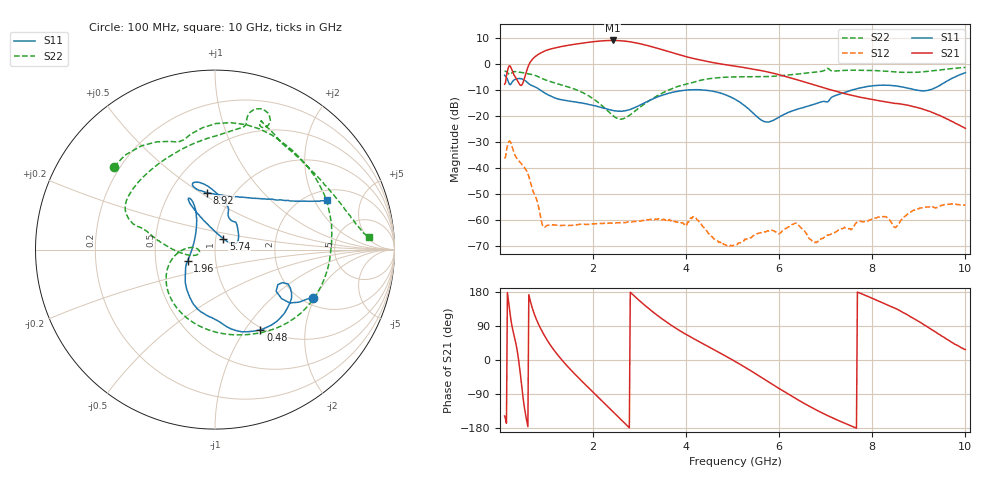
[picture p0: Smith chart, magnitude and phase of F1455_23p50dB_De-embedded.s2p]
! Integrated Device Technology
! Corporate Headquarters
! 6024 Silver Creek Valley Road
! San Jose, CA 95138  USA
! Phone:  1-408-284-8200
! Toll Free:  1-800-223-1366
! Webpage:  http://www.idt.com/
! Timing and RF Division
! 515 Groton Road, Suite 102
! Westford, MA 01886-6024
! Device:  F1455
! Description: 6-bit 0.5 dB Transmit Variable Gain Amplifier
! Frequency:  1400.0 -  2300.00 MHz
! Package:  6x6 mm Thin QFN Plastic Package: 28 pin
! State:  47
! Atten State:  23.5 dB
! Voltage:  +5.00 Volts
! Current:  217.630 mA
! Data:  The device was measured on a the F1455 evaluation board which has
!  individual transmission lines to the RF pins.  Data was collected
!  using a calibrated network analyzer.  The evaluation board was
!  de-embedded using a TRL calibration technique.
!  The reference plane is the edge of the package pin.
!  Pin  1 = CSb
!  Pin  2 = DATA
!  Pin  3 = CLK
!  Pin  4 = RSET
!  Pin  5 = GND
!  Pin  6 = RFIN  = Port 1
!  Pin  7 = GND
!  Pin  8 = NC
!  Pin  9 = NC
!  Pin 10 = NC
!  Pin 11 = NC
!  Pin 12 = NC
!  Pin 13 = NC
!  Pin 14 = /STBY
!  Pin 15 = GND
!  Pin 16 = RFOUT  = Port 2
!  Pin 17 = GND
!  Pin 18 = NC
!  Pin 19 = NC
!  Pin 20 = NC
!  Pin 21 = GND
!  Pin 22 = NC
!  Pin 23 = GND
!  Pin 24 = NC
!  Pin 25 = NC
!  Pin 26 = NC
!  Pin 27 = GND
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# GHz S dB R 50
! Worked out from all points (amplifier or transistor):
!   496 points, 100 MHz to 10 GHz, reference 50 ohm
!   highest |S21| = 9.1 dB at 2.42 GHz (marker M1)
!   |S21| within 3 dB of that: 1.154 GHz to 3.38 GHz (2.226 GHz wide, 98.2 % of centre)
!   unconditionally stable (mu >= 1): start of sweep to end of sweep
!   at 1.74 GHz: K = 212.90, MAG = 8.5 dB, |S12| = -61.6 dB
!   at 5.06 GHz: K = 1073.78, MAG = 1.0 dB, |S12| = -69.6 dB
!   at 10 GHz: K = 614.63, MAG = -16.1 dB, |S12| = -54.3 dB
!   S11 on the Smith chart (normalised r, x): 100 MHz: 2.26, -1.93; 480 MHz: 0.97, -1.18; 1.96 GHz: 0.73, -0.09; 5.74 GHz: 1.09, +0.13; 8.92 GHz: 0.75, +0.53; 10 GHz: 2.45, +2.53
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0.1  -4.31 -26.2  -7.78 -147.9  -36.35 47.2  -2.75 140.7
0.18  -6.73 -36.4  -1.37 160.1  -30.24 -6.9  -3.70 112.6
0.26  -6.95 -25.2  -2.38 88.4  -31.74 -76.9  -3.32 95.9
0.38  -5.60 -42.4  -6.48 17.5  -36.70 -117.8  -3.02 58.0
0.48  -5.78 -60.5  -7.80 -82.6  -38.81 -149.5  -3.29 31.8
0.66  -8.07 -88.2  1.00 152.1  -45.90 141.5  -3.93 -10.1
0.8  -9.21 -106.0  3.45 102.1  -52.80 112.6  -4.68 -41.3
0.96  -11.11 -123.5  5.01 63.6  -62.83 127.5  -5.98 -70.8
1.34  -13.79 -143.6  6.81 -1.3  -62.12 106.5  -8.12 -121.1
1.76  -14.98 -153.5  8.03 -55.9  -61.66 75.9  -10.83 -157.6
1.96  -15.73 -158.2  8.51 -80.0  -61.48 66.8  -12.82 -171.0
2.42  -17.83 179.3  9.09 -135.5  -61.25 49.1  -19.74 176.2
2.82  -17.30 142.7  8.49 176.5  -60.79 39.2  -19.26 -164.1
3.1  -14.98 125.1  7.43 145.5  -60.13 32.8  -15.44 -171.6
3.4  -12.54 116.9  5.98 116.1  -59.53 20.5  -12.04 177.7
4.08  -9.93 116.3  2.47 61.9  -59.66 8.6  -7.38 163.4
5.06  -13.62 114.7  -0.83 -4.3  -69.56 14.2  -4.93 148.4
5.74  -22.27 52.3  -2.97 -55.3  -64.31 19.5  -4.82 120.2
6.7  -15.79 37.1  -7.74 -125.6  -68.03 -139.0  -3.23 78.6
8.36  -8.18 108.6  -14.81 143.3  -59.68 75.3  -2.84 62.6
8.92  -9.88 97.8  -16.51 107.5  -56.12 97.0  -3.16 40.1
10  -3.34 24.0  -24.76 27.7  -54.29 24.9  -1.28 4.7
